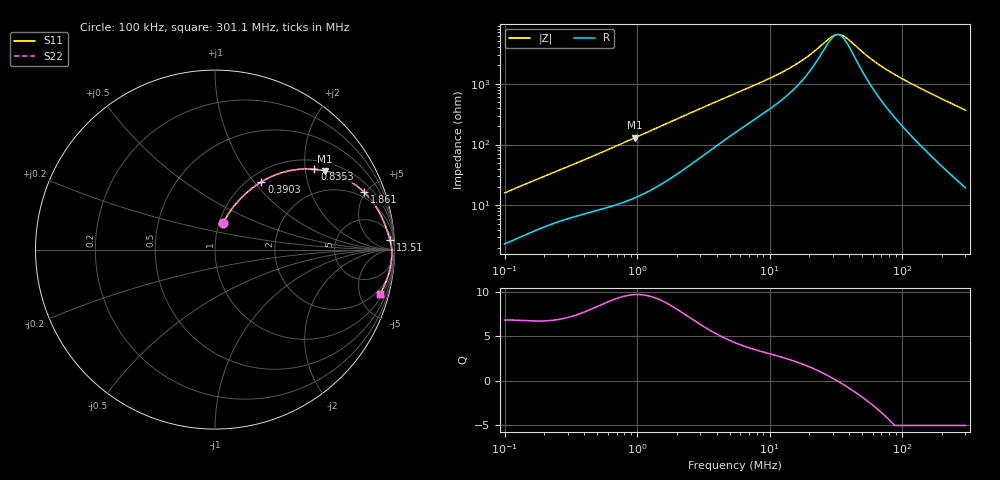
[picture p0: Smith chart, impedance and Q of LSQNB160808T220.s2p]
! LSQNB160808T220  S-PARAMETER MODEL  ( General Type )
! Model Generated by TAIYO YUDEN Corporation (http://www.ty-top.com)
! Version 2.0
! TAIYO YUDEN Control No. 100810NF25SB-FKC
! Copyright(c) 2007 TAIYO YUDEN CO.,LTD. All Rights Reserved.
! Product Description (link to TY-COMPAS)
! https://ds.yuden.co.jp/TYCOMPAS/or/detail?pn=LSQNB160808T220K&u=M
! Products Name : Inductors
! Characteristics :
!  Inductance : 22 uH , SRF(min) : 16 MHz , DC Resistance(max) : 1.3 Ohm
!  Rated Current : Saturation :70 mA , Temp Rise : 230 mA (40 degC)
!  Case Size : 1.6 x 0.8 / 0.063 x 0.031 [mm/inch] , Thickness : 0.8 / 0.031 [mm/inch]
!  (Conditions: Temperature = 25 degC , DC Bias Current/Voltage = 0A / 0V)
! External Node Assignments :
!  1  o---GGG---o  2
! GND o---------o GND
! Frequency Range : 0.1MHz  -  301.082333MHz  [ 402 STEP ]
# MHz S RI R 50
! Freq[MHz].  S11 Real  S11 Imag  S21 Real  S21 Imag  S12 Real  S12 Imag  S22 Real  S22 Imag
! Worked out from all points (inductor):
!   401 points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, 100 kHz to 301.1 MHz, reference 50 ohm
!   read as one part in series: L = 24.7 uH near 104.1 kHz
!   highest Q = 9.68 at 961 kHz (marker M1), where L = 21.3 uH
!   self-resonance near 32.51 MHz
!   S11 on the Smith chart (normalised r, x): 100 kHz: 1.05, +0.32; 390.3 kHz: 1.14, +1.09; 835.3 kHz: 1.23, +2.24; 1.861 MHz: 1.59, +4.88; 13.51 MHz: 14, +32; 301.1 MHz: 1.39, -7.36
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0.1  0.0455 0.1476  0.9545 -0.1476  0.9545 -0.1476  0.0455 0.1476
0.209787  0.1216 0.2611  0.8784 -0.2611  0.8784 -0.2611  0.1216 0.2611
0.382543  0.2522 0.3736  0.7478 -0.3736  0.7478 -0.3736  0.2522 0.3736
0.39028  0.2581 0.3772  0.7419 -0.3772  0.7419 -0.3772  0.2581 0.3772
0.594302  0.408 0.4381  0.592 -0.4381  0.592 -0.4381  0.408 0.4381
0.835318  0.5537 0.4476  0.4463 -0.4476  0.4463 -0.4476  0.5537 0.4476
0.961012  0.6135 0.438  0.3865 -0.438  0.3865 -0.438  0.6135 0.438
1.463388  0.7673 0.3715  0.2327 -0.3715  0.2327 -0.3715  0.7673 0.3715
1.860888  0.8305 0.3199  0.1695 -0.3199  0.1695 -0.3199  0.8305 0.3199
2.949474  0.9058 0.2243  0.0942 -0.2243  0.0942 -0.2243  0.9058 0.2243
5.487097  0.9501 0.1304  0.0499 -0.1304  0.0499 -0.1304  0.9501 0.1304
9.422234  0.968 0.0782  0.032 -0.0782  0.032 -0.0782  0.968 0.0782
13.51122  0.9758 0.052  0.0242 -0.052  0.0242 -0.052  0.9758 0.052
20.99048  0.9819 0.0248  0.0181 -0.0248  0.0181 -0.0248  0.9819 0.0248
29.50303  0.9843 0.00547  0.0157 -0.00547  0.0157 -0.00547  0.9843 0.00547
31.96343  0.9847 0.000964  0.0153 -0.000964  0.0153 -0.000964  0.9847 0.000964
34.62902  0.9849 -0.00356  0.0151 0.00356  0.0151 0.00356  0.9849 -0.00356
39.04995  0.9852 -0.0105  0.0148 0.0105  0.0148 0.0105  0.9852 -0.0105
59.46364  0.9847 -0.0367  0.0153 0.0367  0.0153 0.0367  0.9847 -0.0367
80.29753  0.9827 -0.0591  0.0173 0.0591  0.0173 0.0591  0.9827 -0.0591
146.4211  0.9712 -0.1213  0.0288 0.1213  0.0288 0.1213  0.9712 -0.1213
301.0823  0.9202 -0.2458  0.0798 0.2458  0.0798 0.2458  0.9202 -0.2458
